FUNCTION_BLOCK FB_LN_IED_LD1_XCBR1 EXTENDS FB_AcsiCommonLogicalNodeClass
VAR_INPUT
	NamPlt: FB_DO_IED_LD1_XCBR1_NamPlt := (sClass:='LPL', bLinkResult:=THIS^.AddDataToContainer(ipData:=NamPlt));
	Beh: FB_DO_IED_LD1_XCBR1_Beh := (sClass:='ENS', bLinkResult:=THIS^.AddDataToContainer(ipData:=Beh));
	Health: FB_DO_IED_LD1_XCBR1_Health := (sClass:='ENS', bLinkResult:=THIS^.AddDataToContainer(ipData:=Health));
	Mod_: FB_DO_IED_LD1_XCBR1_Mod := (sObjectName:='Mod', sClass:='ENC', bLinkResult:=THIS^.AddDataToContainer(ipData:=Mod_));
	Loc: FB_DO_IED_LD1_XCBR1_Loc := (sClass:='SPS', bLinkResult:=THIS^.AddDataToContainer(ipData:=Loc));
	OpCnt: FB_DO_IED_LD1_XCBR1_OpCnt := (sClass:='INS', bLinkResult:=THIS^.AddDataToContainer(ipData:=OpCnt));
	Pos: FB_DO_IED_LD1_XCBR1_Pos := (sClass:='DPC', bLinkResult:=THIS^.AddDataToContainer(ipData:=Pos));
	BlkOpn: FB_DO_IED_LD1_XCBR1_BlkOpn := (sClass:='SPC', bLinkResult:=THIS^.AddDataToContainer(ipData:=BlkOpn));
	BlkCls: FB_DO_IED_LD1_XCBR1_BlkCls := (sClass:='SPC', bLinkResult:=THIS^.AddDataToContainer(ipData:=BlkCls));
END_VAR
VAR
END_VAR

END_FUNCTION_BLOCK
